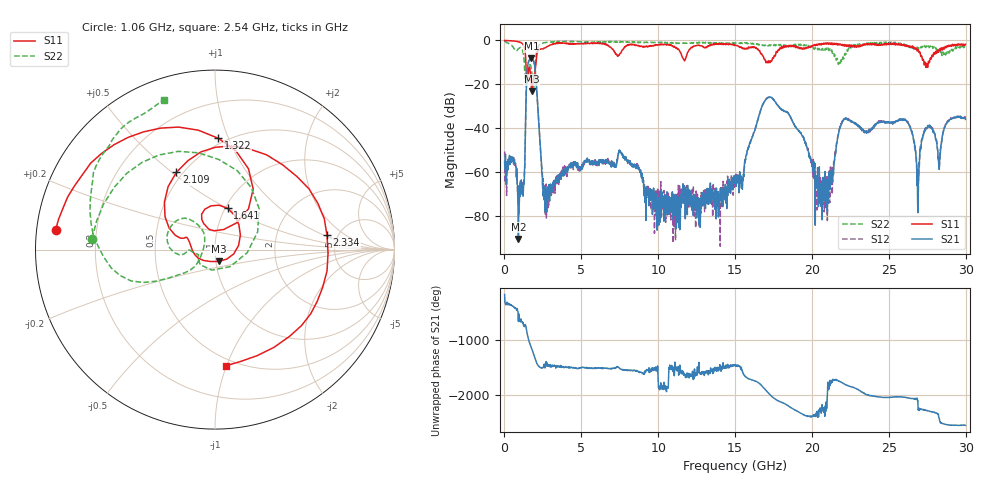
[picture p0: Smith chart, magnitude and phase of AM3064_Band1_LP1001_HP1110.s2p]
# Hz S DB R 50.0
!freq dBS11 angS11 dBS21 angS21 dBS12 angS12 dBS22 angS22
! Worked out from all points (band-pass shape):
!   1600 points, 10 MHz to 29.98 GHz, reference 50 ohm
!   highest |S21| = -8.18 dB at 1.753 GHz (marker M1); lowest = -90.4 dB at 909.7 MHz (marker M2)
!   |S21| within 3 dB of the highest: 1.519 GHz to 1.953 GHz (433.4 MHz wide, 25 % of centre)
!   lowest |S11| = -23.2 dB at 1.772 GHz (marker M3), VSWR 1.15, Z = 51.7 - j6.84 ohm
!   |S11| at or under -10 dB: 1.392 GHz to 2.047 GHz (654.6 MHz wide, 38.1 % of centre); 27.28297 GHz to 27.3521 GHz (69.13 MHz wide, 0.253 % of centre); 27.36 GHz to 27.57 GHz (208.6 MHz wide, 0.759 % of centre)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
!   |S22| runs from -23.7 to -0.4 dB; largest |S21 - S12| = 0.0045
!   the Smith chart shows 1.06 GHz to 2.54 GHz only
!   S11 on the Smith chart (normalised r, x): 1.06 GHz: 0.06, +0.06; 1.322 GHz: 0.46, +0.92; 1.641 GHz: 1.03, +0.50; 2.109 GHz: 0.46, +0.52; 2.334 GHz: 4.09, +1.08; 2.54 GHz: 0.44, -0.99
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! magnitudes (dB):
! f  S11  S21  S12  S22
! 10 MHz  -0.1  -55.3  -50.5  -0.4
! 909.7 MHz  -0.7  -90.4  -69.5  -3.8
! 1.06 GHz  -1.0  -66.7  -68.8  -3.2
! 1.322 GHz  -4.2  -56.6  -56.6  -14.9
! 1.641 GHz  -12.4  -8.8  -8.7  -11.1
! 1.753 GHz  -21.5  -8.2  -8.1  -13.1
! 1.772 GHz  -23.2  -8.2  -8.2  -14.2
! 2.109 GHz  -6.3  -23.6  -23.5  -4.6
! 2.334 GHz  -4.0  -48.1  -49.0  -1.7
! 2.54 GHz  -3.7  -68.5  -66.7  -1.1
! 5.015 GHz  -1.3  -57.8  -58.2  -0.7
! 7.582 GHz  -5.6  -51.2  -51.1  -0.6
! 10 GHz  -2.0  -82.9  -68.1  -0.9
! 15 GHz  -2.2  -62.2  -63.6  -1.4
! 17.2 GHz  -9.2  -26.1  -25.9  -2.2
! 19.99 GHz  -2.9  -56.1  -55.8  -3.0
! 20.93 GHz  -1.4  -73.1  -71.1  -3.6
! 22.07 GHz  -2.0  -36.2  -36.3  -8.4
! 25 GHz  -1.3  -37.0  -37.2  -1.1
! 26.87 GHz  -4.6  -72.3  -64.8  -3.1
! 27.49 GHz  -10.9  -40.1  -39.2  -3.1
! 29.98 GHz  -1.8  -36.0  -35.0  -3.2
